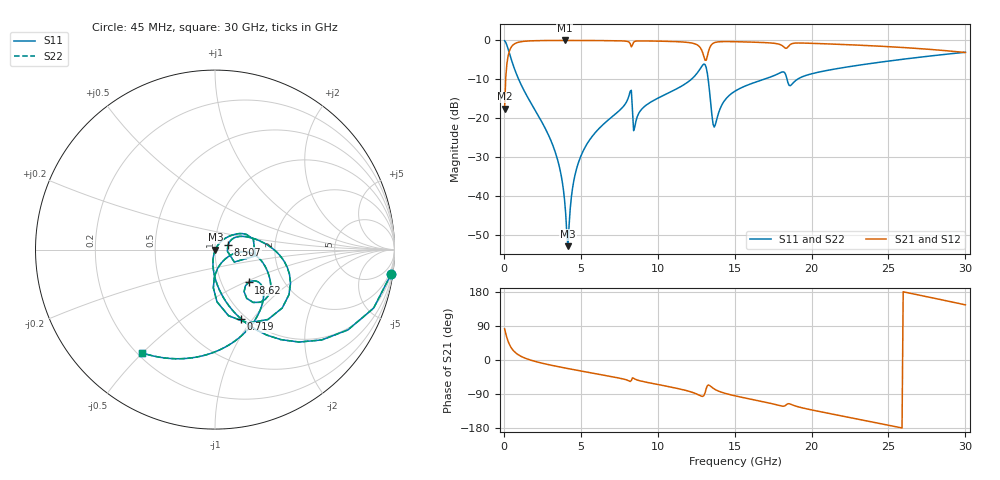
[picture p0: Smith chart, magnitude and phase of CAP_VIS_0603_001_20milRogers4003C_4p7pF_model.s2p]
! S-parameter model data by Modelithics Inc.  support@modelithics.com  813-866-6335  Tampa FL USA
! S-Parameter data specifications:
! Substrate: 20-mil Rogers 4003C, substrate thickness, H=0.508mm, Dielectric constant, Er=3.75
! PCB Mounting Pad Footprint: Pad width, PadW=0.90mm , Pad length, PadL=1.00mm , Pad gap, PadG (edge-to-edge)=1.00mm , Reference planes=3.0mm apart
! Created Wed Nov 18 13:22:57 2015
# hz S ma R 50
! 2 Port Network Data from SP1.SP block
! freq  magS11  angS11  magS21  angS21  magS12  angS12  magS22  angS22
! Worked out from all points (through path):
!   401 points, 45 MHz to 30 GHz, reference 50 ohm
!   highest |S21| = -0.02 dB at 3.939 GHz (marker M1); lowest = -17.6 dB at 45 MHz (marker M2)
!   group delay of S21, straight-line fit = 20.8 ps
!   lowest |S11| = -52.9 dB at 4.164 GHz (marker M3), VSWR 1.00, Z = 50.2 - j0.0304 ohm
!   |S11| at or under -10 dB: 957.9 MHz to 12.19 GHz (11.23 GHz wide, 171 % of centre); 13.28 GHz to 16.91 GHz (3.634 GHz wide, 24.1 % of centre); 18.41 GHz to 19.08 GHz (673.2 MHz wide, 3.59 % of centre)
!   |S22| runs from -52.9 to -0.1 dB; largest |S21 - S12| = 0
!   S11 on the Smith chart (normalised r, x): 45 MHz: 1, -15; 719 MHz: 0.94, -0.88; 8.507 GHz: 1.15, +0.06; 18.62 GHz: 1.34, -0.53; 30 GHz: 0.22, -0.50
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4.5e7  0.9912 -7.9  0.1325 82.1  0.1325 82.1  0.9912 -7.9
3.4455e8  0.6963 -47.7  0.7172 42.3  0.7172 42.3  0.6963 -47.7
7.189875e8  0.4137 -69.3  0.9095 20.5  0.9095 20.5  0.4137 -69.3
3.190275e9  0.0442 -102.3  0.9969 -14.8  0.9969 -14.8  0.0442 -102.3
3.6396e9  0.02211 -103.2  0.9974 -18.5  0.9974 -18.5  0.02211 -103.2
3.93915e9  0.009019 -97.3  0.9975 -20.9  0.9975 -20.9  0.009019 -97.3
4.163812e9  0.002262 -7.7  0.9975 -22.6  0.9975 -22.6  0.002262 -7.7
4.613138e9  0.01829 56.7  0.9971 -26.0  0.9971 -26.0  0.01829 56.7
5.062462e9  0.0347 56.5  0.9965 -29.4  0.9965 -29.4  0.0347 56.5
8.13285e9  0.1948 25.6  0.9491 -55.1  0.9491 -55.1  0.1948 25.6
8.507288e9  0.07682 19.5  0.97 -50.2  0.97 -50.2  0.07682 19.5
1.007992e10  0.1837 23.3  0.9771 -65.2  0.9771 -65.2  0.1837 23.3
1.225166e10  0.3248 0.5  0.9213 -85.3  0.9213 -85.3  0.3248 0.5
1.300054e10  0.4961 -41.0  0.6176 -93.9  0.6176 -93.9  0.4961 -41.0
1.337498e10  0.2137 -92.5  0.8012 -67.4  0.8012 -67.4  0.2137 -92.5
1.374941e10  0.08298 -28.7  0.943 -78.3  0.943 -78.3  0.08298 -28.7
1.50225e10  0.2225 -7.6  0.9618 -94.5  0.9618 -94.5  0.2225 -7.6
1.809289e10  0.3929 -41.2  0.8556 -121.8  0.8556 -121.8  0.3929 -41.2
1.86171e10  0.2614 -44.4  0.8856 -116.3  0.8856 -116.3  0.2614 -44.4
2.003996e10  0.3735 -43.5  0.916 -132.0  0.916 -132.0  0.3735 -43.5
2.505742e10  0.5437 -83.4  0.8291 -172.6  0.8291 -172.6  0.5437 -83.4
3e10  0.7036 -125.1  0.6981 145.6  0.6981 145.6  0.7036 -125.1
